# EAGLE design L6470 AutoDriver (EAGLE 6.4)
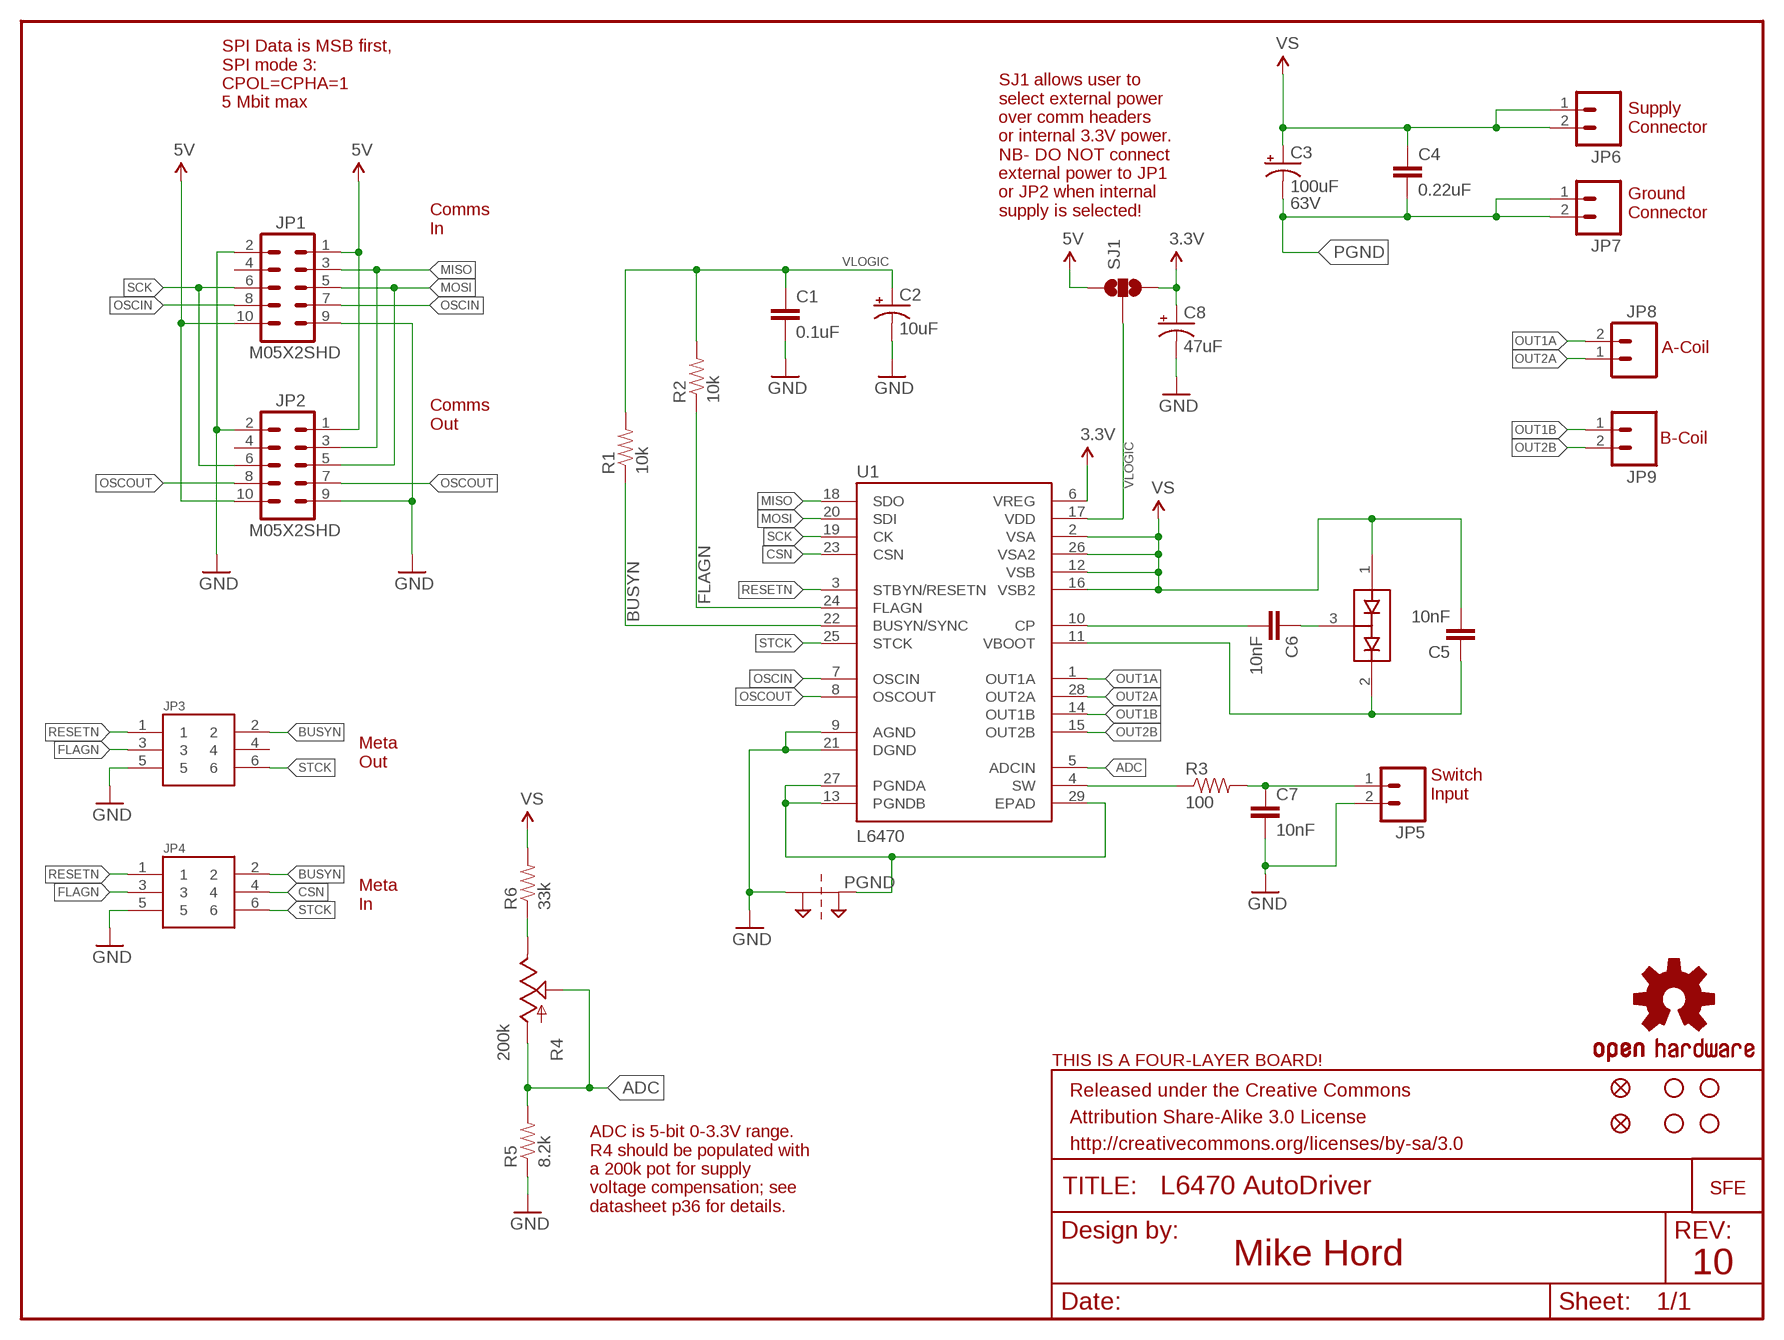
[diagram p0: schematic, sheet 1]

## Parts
C1  0.1uF  .1UF-CER  [0402-CAP]
C2  10uF  10UF-TANT  [EIA3216]
C3  100uF  100UF-ELECT  [PANASONIC_H13]
C4  0.22uF  .22UF-CER  [0402-CAP]
C5  10nF  10NF-CER  [0402-CAP]
C6  10nF  10NF-CER  [0402-CAP]
C7  10nF  10NF-CER  [0402-CAP]
C8  47uF  47UF-TANT  [EIA3528]
D1  BAV99  [SOT23]
FID1  FIDUCIALUFIDUCIAL  [MICRO-FIDUCIAL]
FID2  FIDUCIALUFIDUCIAL  [MICRO-FIDUCIAL]
FRAME1  FRAME-LETTER  [CREATIVE_COMMONS]
JP1  M05X2SHD  [2X5-SHROUDED]
JP2  M05X2SHD  [2X5-SHROUDED]
JP3  M03X2  [2X3-SHROUDED]
JP4  M03X2  [2X3-SHROUDED]
JP5  M023.5MM  [SCREWTERMINAL-3.5MM-2]
JP6  M023.5MM  [SCREWTERMINAL-3.5MM-2]
JP7  M023.5MM  [SCREWTERMINAL-3.5MM-2]
JP8  M023.5MM  [SCREWTERMINAL-3.5MM-2]
JP9  M023.5MM  [SCREWTERMINAL-3.5MM-2]
LOGO1  OSHW-LOGOS  [OSHW-LOGO-S]
LOGO2  LOGO-SFENEW  [SFE-NEW-WEBLOGO]
R1  10k  10K-1%RES-00824  [0402-RES]
R2  10k  10K-1%RES-00824  [0402-RES]
R3  100  100-1%  [0402-RES]
R4  200k  POT100K_3362U  [3362U]
R5  8.2k  8.2K-5%  [0402-RES]
R6  33k  33K-1%  [0402-RES]
SJ1  SOLDERJUMPER_2WAYPASTE1&2  [SJ_3_PASTE1&2]
SJ2  2PT_GND_TIE  [2PT_GND_TIE]
STANDOFF1  STAND-OFF  [STAND-OFF]
STANDOFF2  STAND-OFF  [STAND-OFF]
STANDOFF3  STAND-OFF  [STAND-OFF]
STANDOFF4  STAND-OFF  [STAND-OFF]
U1  L6470  L6470  [HTSSOP28]
U$4  FOUR_LAYER_WARNING  [FOUR_LAYER_WARNING]

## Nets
3.3V: C8.A(+) SJ1.3 U1.6(VREG)
5V: JP1.1 JP1.10 JP2.1 JP2.10 SJ1.1
ADC: R4.P$2(S) R4.P$3(A) R5.2 U1.5(ADCIN)
BUSYN: JP3.2 JP4.2 R1.1 U1.22(BUSYN/SYNC)
CSN: JP4.4 U1.23(CSN)
FLAGN: JP3.3 JP4.3 R2.1 U1.24(FLAGN)
GND: C1.2 C2.C(-) C7.2 C8.C(-) JP1.2 JP1.9 JP2.2 JP2.9 JP3.5 JP4.5 JP5.2 R5.1 SJ2.P$1 U1.9(AGND) U1.21(DGND)
MISO: JP1.3 JP2.3 U1.18(SDO)
MOSI: JP1.5 JP2.5 U1.20(SDI)
N$5: R3.1 U1.4(SW)
N$6: C7.1 JP5.1 R3.2
N$7: C6.2 U1.10(CP)
N$8: C6.1 D1.3(COM)
N$9: C5.1 D1.2(C2) U1.11(VBOOT)
N$11: R4.P$1(E) R6.1
OSCIN: JP1.7 JP1.8 U1.7(OSCIN)
OSCOUT: JP2.7 JP2.8 U1.8(OSCOUT)
OUT1A: JP8.2 U1.1(OUT1A)
OUT1B: JP9.1 U1.14(OUT1B)
OUT2A: JP8.1 U1.28(OUT2A)
OUT2B: JP9.2 U1.15(OUT2B)
PGND: C3.- C4.2 JP7.1 JP7.2 SJ2.P$2 U1.13(PGNDB) U1.27(PGNDA) U1.29(EPAD)
RESETN: JP3.1 JP4.1 U1.3(STBYN/RESETN)
SCK: JP1.6 JP2.6 U1.19(CK)
STCK: JP3.6 JP4.6 U1.25(STCK)
VLOGIC: C1.1 C2.A(+) R1.2 R2.2 SJ1.2 U1.17(VDD)
VS: C3.+ C4.1 C5.2 D1.1(A1) JP6.1 JP6.2 R6.2 U1.2(VSA) U1.12(VSB) U1.16(VSB2) U1.26(VSA2)
Unconnected: JP1.4 JP2.4 JP3.4

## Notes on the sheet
- SPI Data is MSB first,
  SPI mode 3:
  CPOL=CPHA=1
  5 Mbit max
- Supply
  Connector
- 63V
- SJ1 allows user to
  select external power
  over comm headers
  or internal 3.3V power.
  NB- DO NOT connect
  external power to JP1
  or JP2 when internal
  supply is selected!
- Ground
  Connector
- Comms
  In
- A-Coil
- Comms
  Out
- B-Coil
- Meta
  Out
- Switch
  Input
- Meta
  In
- ADC is 5-bit 0-3.3V range.
  R4 should be populated with
  a 200k pot for supply
  voltage compensation; see
  datasheet p36 for details.
- Mike Hord | 10

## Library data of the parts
C1 = SparkFun-Capacitors:.1UF-CER: .1uF ceramic SMT; PROD_ID: CAP-00810
C2 = SparkFun-Capacitors:10UF-TANT: 10uF Tantalum SMT; PROD_ID: CAP-00811
C3 = SparkFun-Capacitors:100UF-ELECT: 100uF electrolytic SMT; PROD_ID: CAP-08362
C4 = SparkFun-Capacitors:.22UF-CER: .22uF ceramic SMT; PROD_ID: CAP-09885; VALUE: .22uF
C5-C7 = SparkFun-Capacitors:10NF-CER: 10nF/.01uF/10000pF ceramic SMT; PROD_ID: CAP-00867
C8 = SparkFun-Capacitors:47UF-TANT: 47uF Tantalum SMT; PROD_ID: CAP-08310
D1 = SparkFun-DiscreteSemi:BAV99: Two small signal silicon diodes connected anode to cathode. Connections to all three nodes available. DIO-10647; PROD_ID: DIO-10647
FID1 FID2 = SparkFun-Aesthetics:FIDUCIAL: Fiducial Alignment Points
FRAME1 = SparkFun-Aesthetics:FRAME-LETTER: Schematic Frame
JP1 JP2 = SparkFun-Connectors:M05X2: Header 5x2 Standard 10-pin dual row 0.1" header. Commonly used with AVR-ISP. Use with Spark Fun Electronics SKU: PRT-00778
JP3 JP4 = SparkFun-Connectors:M03X2: Shrouded 2x3 .1" header, with keying.
JP5-JP9 = SparkFun:M02: Header 2
LOGO1 = SparkFun:OSHW-LOGO: Open Source Hardware Logo This logo indicates the piece of hardware it is found on incorporates a OSHW license and/or adheres to the definition of open source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
LOGO2 = SparkFun:LOGO-SFE: Spark Fun Electronics PCB Logo
R1 R2 = SparkFun-Resistors:10K-1%: 10k-ohm SMT; PROD_ID: RES-00824
R3 = SparkFun-Resistors:100-1%: 100-ohm SMT; PROD_ID: RES-07863
R4 = SparkFun:POT
R5 = SparkFun-Resistors:8.2K-5%: 8.2k-ohm SMT; PROD_ID: RES-10646
R6 = SparkFun-Resistors:33K-1%: 33k-ohm SMT; PROD_ID: RES-08416
SJ1 = SparkFun-Passives:SOLDERJUMPER_2WAY: Solder Jumper 2 way solder jumper
SJ2 = SparkFun-Passives:2PT_GND_TIE: Package for connecting two ground nets in one place.
STANDOFF1-STANDOFF4 = SparkFun:STAND-OFF: Stand Off
U1 = SparkFun-PowerIC:L6470: 3A RMS/7A peak bipolar stepper motor driver with SPI control and step input in HTSSOP-28 package. IC-10648; PROD_ID: IC-10648
U$4 = SparkFun-Aesthetics:FOUR_LAYER_WARNING: Warning text which will appear on both the schematic

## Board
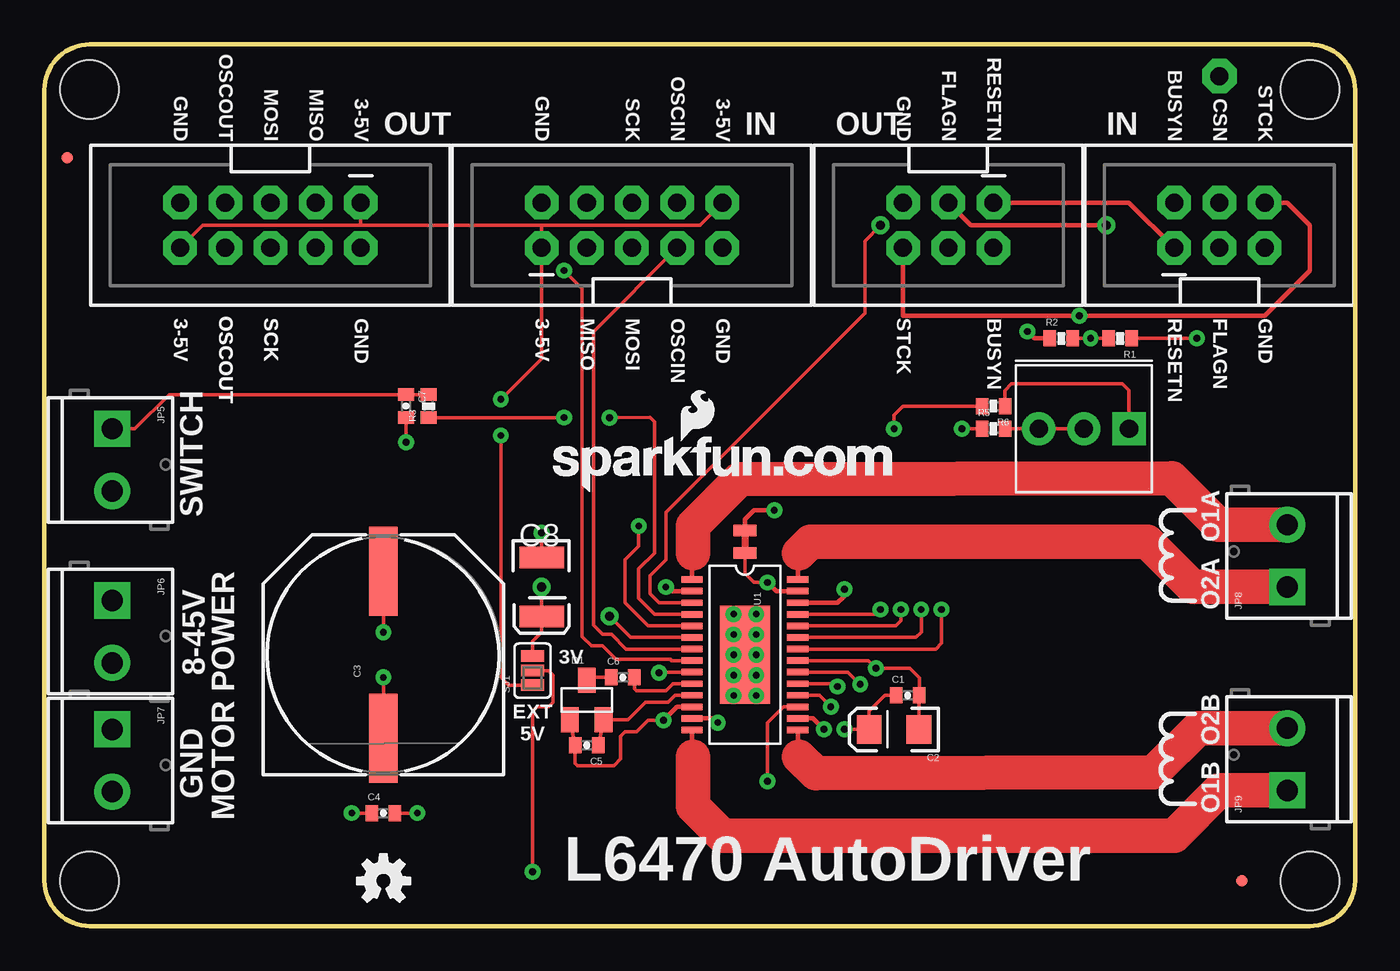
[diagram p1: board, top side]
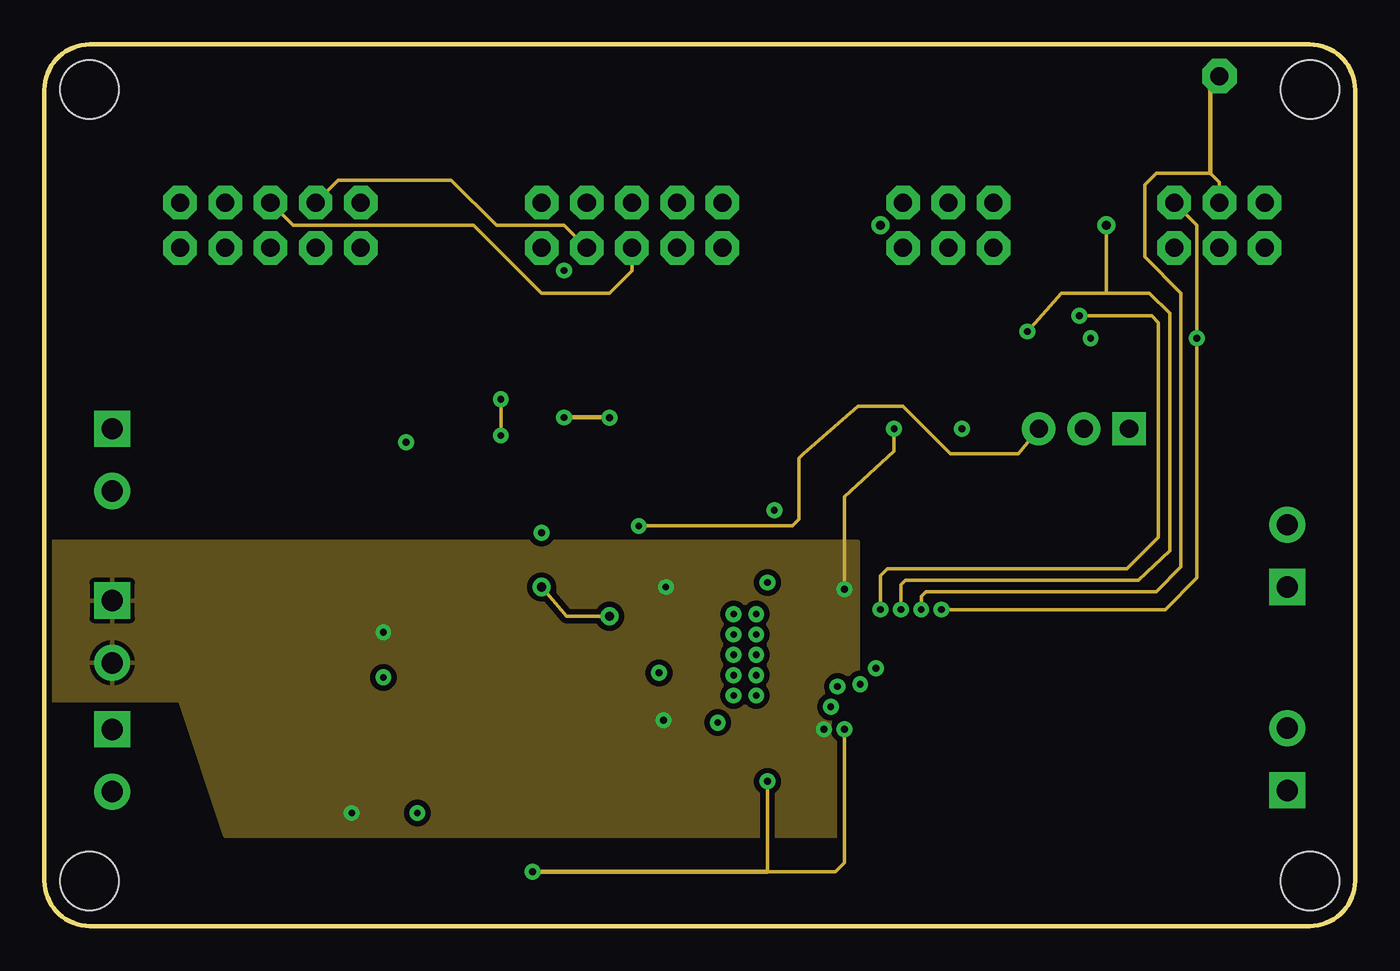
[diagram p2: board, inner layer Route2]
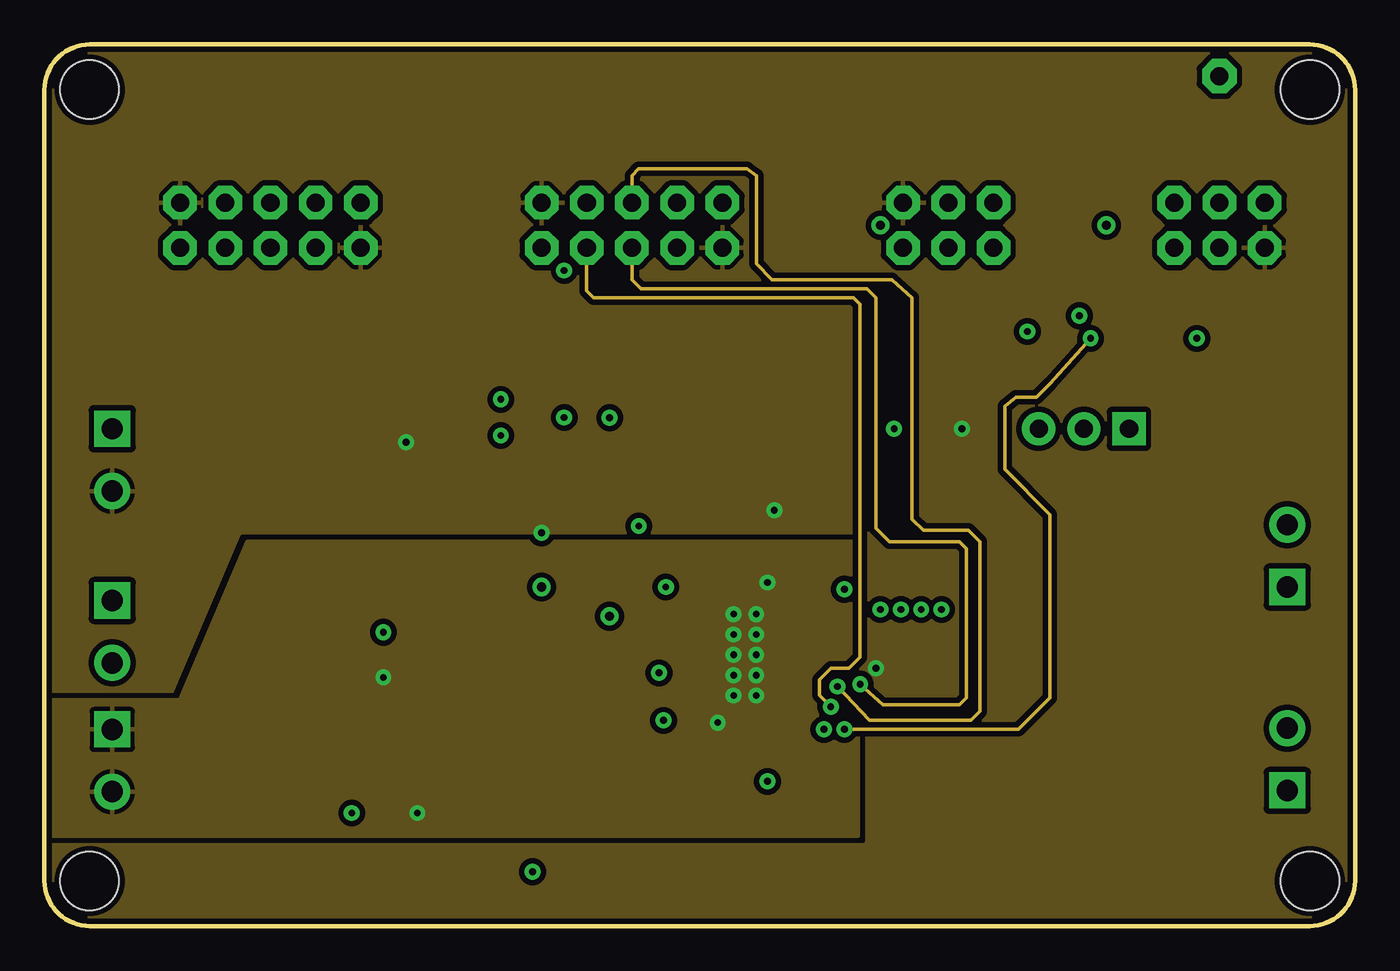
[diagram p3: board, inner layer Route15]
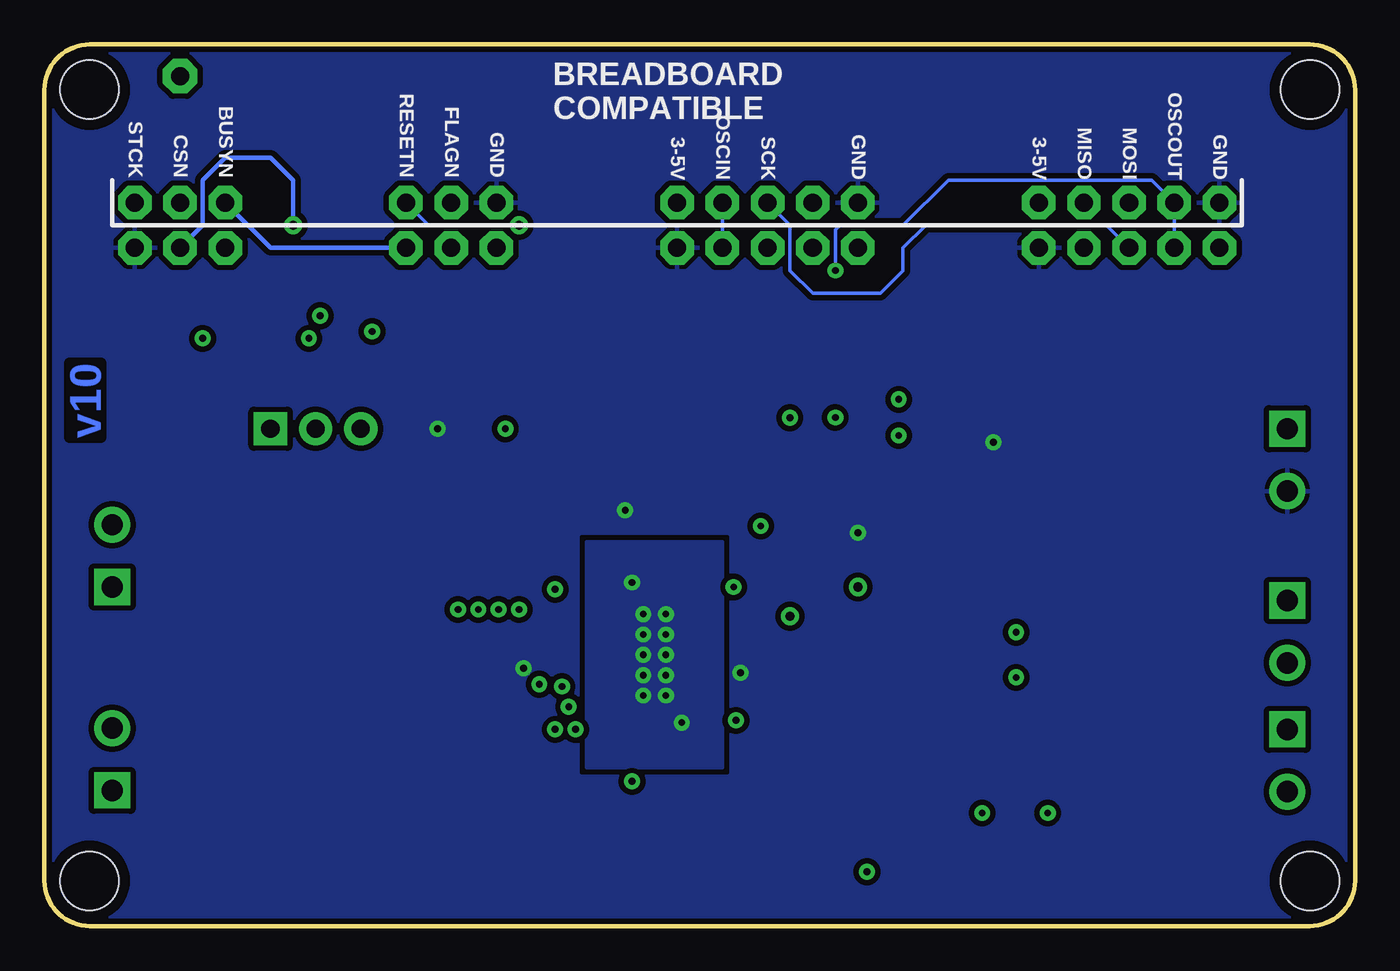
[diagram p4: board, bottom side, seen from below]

Size 73.66 x 49.53 mm. Coordinates in mm from the lower left corner, seen from the top.
Outline: 71.12,0 2.54,0 arc-90 0,2.54 0,46.99 arc-90 2.54,49.53 71.12,49.53 arc-90 73.66,46.99 73.66,2.54 arc-90 71.12,0
Copper layers (1*2*15*16): Top 0.035mm / dielectric 1.5mm / Route2 0.035mm / dielectric 0.15mm / Route15 0.035mm / dielectric 0.2mm / Bottom 0.035mm
Design rules "default": minimum track width 8mil, minimum drill 15mil, track to track 8mil, track to pad 8mil, pad to pad 8mil, via to via 8mil, smd to smd 8mil, copper to edge 8mil, drill to drill 8mil, minimum pad ring 12mil, minimum via ring 10mil, stop-mask expansion 4mil, vias tented up to drill 20mil, thermal gap 10mil

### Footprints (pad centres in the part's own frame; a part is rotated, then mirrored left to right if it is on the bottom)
0402-CAP = smd 0.7 x 0.9: 1 -0.65,0; 2 0.65,0
EIA3216 = smd 1.4 x 1.6: A 1.4,0; C -1.4,0
PANASONIC_H13 = smd 5 x 1.6: + 4.7,0; - -4.7,0
EIA3528 = smd 1.2 x 2.5: A 1.65,0; C -1.65,0
SOT23 = smd 1 x 1.4: 1 -0.95,-1.1; 2 0.95,-1.1; 3 0,1.1
MICRO-FIDUCIAL = smd 0.635 x 0.635: 1 0,0
2X5-SHROUDED = drill 1.016 pad 1.88 octagon: 1 -1.27,5.08; 2 1.27,5.08; 3 -1.27,2.54; 4 1.27,2.54; 5 -1.27,0; 6 1.27,0; 7 -1.27,-2.54; 8 1.27,-2.54; 9 -1.27,-5.08; 10 1.27,-5.08
2X3-SHROUDED = drill 1.016 pad 1.88 octagon: 1 -1.27,2.54; 2 1.27,2.54; 3 -1.27,0; 4 1.27,0; 5 -1.27,-2.54; 6 1.27,-2.54
SCREWTERMINAL-3.5MM-2 = drill 1.2 pad 2.032 square: 1 0,0 | drill 1.2 pad 2.032: 2 3.5,0
0402-RES = smd 0.7 x 0.9: 1 -0.65,0; 2 0.65,0
3362U = drill 1.016 pad 1.88 square: P$1 0,2.54 | drill 1.016 pad 1.88: P$2 2.54,2.54; P$3 5.08,2.54
SJ_3_PASTE1&2 = smd 0.635 x 1.27: 1 -0.813,0; 2 0,0; 3 0.813,0
2PT_GND_TIE = smd 1.27 x 0.635: P$1 0,0.635; P$2 0,-0.635
STAND-OFF = hole 3.302: 0,0
HTSSOP28 = smd 0.36 x 1.19: 1 -4.225,-2.97; 2 -3.575,-2.97; 3 -2.925,-2.97; 4 -2.275,-2.97; 5 -1.625,-2.97; 6 -0.975,-2.97; 7 -0.325,-2.97; 8 0.325,-2.97; 9 0.975,-2.97; 10 1.625,-2.97; 11 2.275,-2.97; 12 2.925,-2.97; 13 3.575,-2.97; 14 4.225,-2.97; 15 4.225,2.97; 16 3.575,2.97; 17 2.925,2.97; 18 2.275,2.97; 19 1.625,2.97; 20 0.975,2.97; 21 0.325,2.97; 22 -0.325,2.97; 23 -0.975,2.97; 24 -1.625,2.97; 25 -2.275,2.97; 26 -2.925,2.97; 27 -3.575,2.97; 28 -4.225,2.97 | smd 5.5 x 2.8: 29 0,0

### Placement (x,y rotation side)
C1  48.51,12.95 0 top
C2  47.75,11.05 180 top
C3  19.05,15.24 90 top
C4  19.05,6.35 0 top
C5  30.48,10.16 180 top
C6  32.51,13.97 0 top
C7  20.32,29.21 270 top
C8  27.94,19.05 270 top
D1  30.48,12.7 0 top
FID1  67.31,2.54 0 top
FID2  1.27,43.18 0 top
FRAME1  not placed on the board
JP1  33.02,39.37 90 top
JP2  12.7,39.37 270 top
JP3  50.8,39.37 270 top
JP4  66.04,39.37 90 top
JP5  3.81,27.94 270 top
JP6  3.81,18.29 270 top
JP7  3.81,11.05 270 top
JP8  69.85,19.05 90 top
JP9  69.85,7.62 90 top
LOGO1  19.05,2.54 0 top
LOGO2  28.57,24.38 0 top
R1  60.45,33.02 180 top
R2  57.15,33.02 0 top
R3  21.59,29.21 90 top
R4  60.96,30.48 180 top
R5  53.34,27.94 0 top
R6  53.34,29.21 180 top
SJ1  27.43,14.35 90 top
SJ2  39.37,21.59 0 top
STANDOFF1  71.12,46.99 0 top
STANDOFF2  71.12,2.54 0 top
STANDOFF3  2.54,2.54 0 top
STANDOFF4  2.54,46.99 0 top
U1  39.37,15.24 270 top
U$4  0,-2.54 0 top

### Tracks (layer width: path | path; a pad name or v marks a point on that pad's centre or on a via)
3.3V  (via drill 0.51)
  Top 0.203: U1.6 32.93,16.21 v31.75,17.4 | v27.94,19.05 C8.A 27.94,16.51 27.43,16 SJ1.3
  Route2 0.203: v27.94,19.05 29.34,17.4 v31.75,17.4
5V  (via drill 0.38)
  Top 0.203: SJ1.1 26.09,13.54 25.65,13.97 v25.65,27.56 | v25.65,29.59 27.94,31.88 JP1.1 27.94,39.37 | JP1.10 36.83,39.37 27.94,39.37 | 27.94,39.37 17.78,39.37 | 17.78,39.37 8.89,39.37 JP2.10 | JP2.1 17.78,39.37
  Route2 0.203: v25.65,27.56 v25.65,29.59
ADC  (via drill 0.38)
  Top 0.203: U1.5 33.94,16.86 32.64,18.16 32.64,20.57 33.4,21.34 v33.4,22.48 | R5.2 R4.P$3 R4.P$2
  Route2 0.203: v33.4,22.48 42.04,22.48 42.42,22.86 42.42,26.29 42.67,26.54 45.72,29.21 48.26,29.21 50.93,26.54 54.74,26.54 R4.P$3
BUSYN  (via drill 0.38)
  Top 0.203: U1.22 50.11,15.56 50.42,15.88 v50.42,17.78 | R1.1 v64.77,33.02
  Route2 0.203: v50.42,17.78 62.99,17.78 64.77,19.56 v64.77,33.02 64.77,39.37 JP4.2
  Bottom 0.254: JP3.2 60.96,38.1 JP4.2
CSN  (via drill 0.38, 1.02 pad 1.93)
  Top 0.203: U1.23 48.98,16.21 49.28,16.51 v49.28,17.78
  Route2 0.203: v49.28,17.78 49.28,18.54 49.53,18.8 62.48,18.8 63.88,20.19 63.88,35.56 61.85,37.59 61.85,41.66 62.48,42.29 65.53,42.29 66.04,41.78 JP4.4
  Route2 0.254: 65.53,42.29 65.53,47.24 v66.04,47.75
FLAGN  (via drill 0.38, 0.51)
  Top 0.203: U1.24 47.85,16.86 48.13,17.14 v48.13,17.78
  Top 0.254: JP3.3 52.07,39.37 v59.69,39.37 | R2.1 55.63,33.02 v55.24,33.4
  Route2 0.203: v48.13,17.78 48.13,19.18 48.39,19.43 61.47,19.43 63.25,21.08 63.25,34.42 62.1,35.56 59.69,35.56 | v55.24,33.4 57.15,35.56 59.69,35.56 | v59.69,39.37 59.69,35.56
  Bottom 0.254: v59.69,39.37 59.69,41.91 60.96,43.18 63.5,43.18 64.77,41.91 64.77,39.37 JP4.3
GND  (via drill 0.38)
  Top 0.203: U1.21 46.3,14.91 v46.74,14.48 48.64,14.48 49.16,13.96 C1.2 C2.C | R5.1 v51.56,27.94 | U1.9 34.59,14.27 v34.54,14.22 | C8.C v27.94,22.1 | C7.2 v20.32,27.18
  Top 0.254: v41.02,23.37 39.88,23.37 39.37,22.86 SJ2.P$1
  pour Route15 (isolate 0.305, rank 2): 71.12,0 2.54,0 arc-90 0,2.54 0,46.99 arc-90 2.54,49.53 71.12,49.53 arc-90 73.66,46.99 73.66,2.54 arc-90
  pour Bottom (isolate 0.305, rank 2): 71.12,0 2.54,0 arc-90 0,2.54 0,46.99 arc-90 2.54,49.53 71.12,49.53 arc-90 73.66,46.99 73.66,2.54 arc-90
MISO  (via drill 0.38)
  Top 0.203: U1.18 43.55,12.96 v44.2,12.32
  Route2 0.203: JP2.3 16.51,41.91 22.86,41.91 25.4,39.37 29.21,39.37 JP1.3
  Route15 0.203: v44.2,12.32 43.56,12.95 43.56,13.84 44.2,14.48 45.21,14.48 45.85,15.11 45.85,34.92 45.47,35.31 30.86,35.31 30.48,35.69 JP1.3
MOSI  (via drill 0.38)
  Top 0.203: U1.20 45.17,14.27 v45.85,13.59
  Route2 0.203: JP2.5 13.97,39.37 24.13,39.37 27.94,35.56 31.75,35.56 33.02,36.83 JP1.5
  Route15 0.203: v45.85,13.59 47.12,12.45 51.44,12.45 51.82,12.83 51.82,21.21 51.44,21.59 47.5,21.59 46.74,22.35 46.74,35.31 46.23,35.81 33.53,35.81 33.02,36.32 JP1.5
N$5  (via drill 0.38)
  Top 0.203: U1.4 34.3,17.52 33.4,18.41 33.4,20.07 34.29,20.95 34.29,28.32 34.04,28.57 v31.77,28.56 | R3.1 29.2,28.56 v29.21,28.57
  Route2 0.254: v29.21,28.57 31.75,28.57 v31.77,28.56
N$6
  Top 0.203: JP5.1 5.08,27.94 7,29.86 C7.1 R3.2
N$7
  Top 0.203: C6.2 33.16,13.32 33.27,13.21 34.92,13.21 35.33,13.62 U1.10
N$8
  Top 0.203: C6.1 30.65,13.97 D1.3
N$9
  Top 0.203: U1.11 35.44,12.96 35.05,12.57 33.78,12.57 32.81,11.6 D1.2 C5.1
N$11
  Top 0.203: R6.1 53.99,30.08 54.36,30.48 60.58,30.48 60.96,30.1 R4.P$1
OSCIN
  Top 0.203: U1.7 32.7,15.56 31.88,16.38 31.37,16.38 30.86,16.89 30.86,33.4 JP1.7
  Bottom 0.203: JP1.7 JP1.8
OSCOUT  (via drill 0.38)
  Top 0.203: U1.8 35.25,14.91 35.18,14.99 32.13,14.99 31.37,15.75 30.73,15.75 30.23,16.26 30.23,35.81 v29.21,36.83
  Bottom 0.203: JP2.8 JP2.7 11.43,41.91 22.86,41.91 25.4,39.37 28.96,39.37 29.21,39.12 v29.21,36.83
OUT1A
  Top 0.254: U1.1 36.4,20.91 36.45,20.95
  Top 1.93: JP8.2 65.97,22.55 63.37,25.15 39.06,25.09 36.45,22.48 36.45,20.95
OUT1B
  Top 0.254: U1.14 36.4,9.57 36.45,9.53
  Top 1.93: JP9.1 66.04,7.62 63.5,5.08 38.1,5.08 36.45,6.73 36.45,9.53
OUT2A
  Top 0.254: U1.28 42.34,20.88 42.42,20.95
  Top 1.93: JP8.1 64.52,19.05 61.98,21.59 43.05,21.59 42.42,20.95
OUT2B
  Top 0.254: U1.15 42.34,9.6 42.42,9.53
  Top 1.93: JP9.2 64.84,11.12 62.36,8.64 43.36,8.58 42.42,9.53
PGND  (via drill 0.38)
  Top 0.203: v40.64,19.3 39.88,19.3 39.37,19.81 SJ2.P$2 | U1.29 v40.01,15.24 | C4.2 v20.95,6.35 | C3.- v19.05,13.97
  Top 0.254: U1.27 41.13,18.82 v40.64,19.3 | U1.13 37.61,11.66 v37.85,11.43
  other vias: 40.01,12.95 38.73,12.95 40.01,14.1 38.73,14.1 38.73,15.24 40.01,16.38 38.73,16.38 40.01,17.53 38.73,17.53
  pour Route15 (isolate 0.305): 0,5.08 45.72,5.08 45.72,21.59 11.43,21.59 7.62,12.7 0,12.7
  pour Bottom (isolate 0.305): 35.56,8.89 35.56,21.59 43.18,21.59 43.18,8.89
RESETN  (via drill 0.51)
  Top 0.203: U1.3 34.54,18.16 34.04,18.67 34.04,19.68 34.92,20.57 34.92,23.24 46.1,34.42 46.1,38.48 v46.99,39.37
  Top 0.254: JP3.1 60.96,40.64 JP4.1
  Bottom 0.203: v46.99,39.37 52.07,39.37 JP3.1
SCK  (via drill 0.38)
  Top 0.203: U1.19 44.42,13.62 v44.58,13.46
  Route15 0.203: v44.58,13.46 46.35,11.56 52.07,11.56 52.58,12.06 52.58,21.59 51.94,22.23 49.4,22.23 48.77,22.86 48.77,35.31 47.62,36.32 40.89,36.32 40.01,37.21 40.01,42.16 39.5,42.55 33.4,42.55 33.02,42.16 JP1.6
  Bottom 0.203: JP2.6 13.97,39.37 24.13,39.37 25.4,38.1 25.4,36.83 26.67,35.56 30.48,35.56 31.75,36.83 31.75,39.37 JP1.6
STCK  (via drill 0.38)
  Top 0.203: U1.25 46.73,17.52 v46.99,17.78
  Top 0.254: JP3.6 48.26,34.29 v58.17,34.29 68.58,34.29 71.12,36.83 71.12,39.37 69.85,40.64 JP4.6
  Route2 0.203: v46.99,17.78 46.99,19.68 47.37,20.07 60.83,20.07 62.61,21.84 62.61,33.91 62.23,34.29 v58.17,34.29
VLOGIC  (via drill 0.38)
  Top 0.203: v44.96,11.05 C2.A 46.35,12.06 47.24,12.95 C1.1 | U1.17 41.52,12.31 40.64,11.43 v40.64,8.13 | v27.43,3.05 27.43,12.06 27.69,12.32 28.32,12.32 28.57,12.57 28.57,14.1 28.32,14.35 SJ1.2 | R2.2 v58.8,33.02 R1.2
  Route2 0.203: v44.96,11.05 44.96,3.56 44.45,3.05 40.64,3.05 v40.64,8.13
  Route2 0.254: 40.64,3.05 v27.43,3.05
  Route15 0.203: v44.96,11.05 54.74,11.05 56.52,12.83 56.52,23.11 53.98,25.65 53.98,29.21 54.61,29.72 55.75,29.72 56.52,30.48 v58.8,33.02
VS  (via drill 0.38)
  Top 0.203: R6.2 48.26,29.21 47.75,28.7 v47.75,27.94 | D1.1 C5.2 29.83,9.16 29.97,9.02 32,9.02 32.38,9.4 32.38,10.67 32.64,10.92 33.27,10.92 33.91,11.56 v34.8,11.56 | C3.+ v19.05,16.51 | C4.1 v17.27,6.35
  Top 0.254: U1.26 44.58,18.16 44.96,18.54 v44.96,18.92 | U1.2 35.16,18.82 v34.92,19.05 | U1.16 43.2,11.66 v43.81,11.05 | U1.12 35.56,12.31 v34.8,11.56
  Route2 0.203: v47.75,27.94 47.75,26.67 44.96,24.13 v44.96,18.92
  pour Route2 (isolate 0.305, rank 3): 0,21.59 45.72,21.59 45.72,5.08 10.16,5.08 7.62,12.7 0,12.7

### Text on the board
Bottom: v10
tPlace: GND | OSCOUT | MOSI | MISO | 3-5V | OUT | GND | SCK | OSCIN | 3-5V | IN | OUT | GND | FLAGN | RESETN | IN | BUSYN | CSN | STCK | 3-5V | OSCOUT | OSCOUT | SCK | SCK | GND | 3-5V | MISO | MOSI | OSCIN | GND | STCK | BUSYN | RESETN | FLAGN | GND | SWITCH | O1A | O2A | 8-45V | 3V | MOTOR POWER | EXT / 5V | O2B | GND | O1B | L6470 AutoDriver
bPlace: BREADBOARD / COMPATIBLE | GND | OSCOUT | MOSI | MISO | 3-5V | GND | SCK | OSCIN | 3-5V | GND | FLAGN | RESETN | BUSYN | CSN | STCK
tValues: M.Hord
